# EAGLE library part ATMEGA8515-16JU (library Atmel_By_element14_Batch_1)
Microcontroller with 8K Bytes In-System Programmable Flash
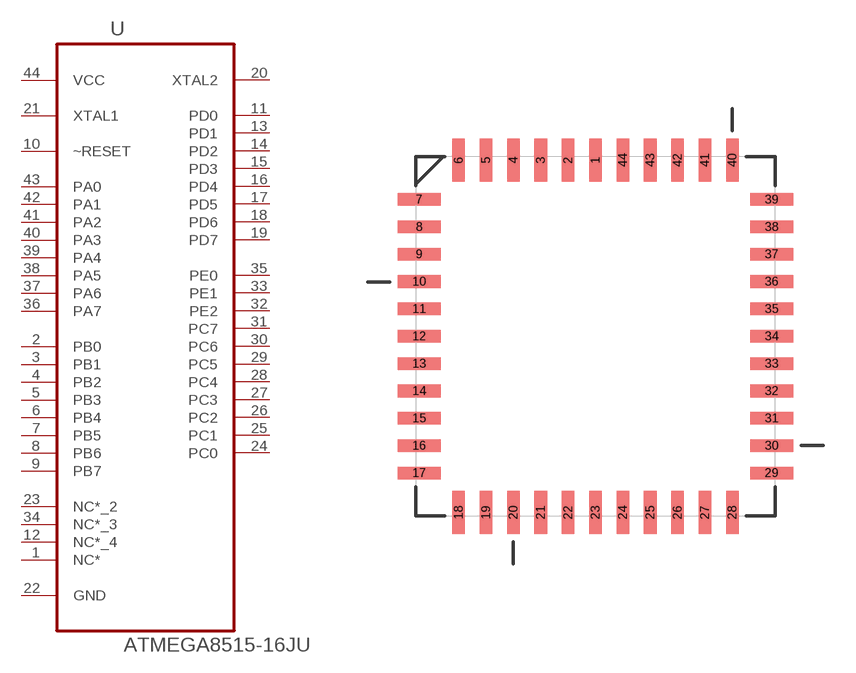
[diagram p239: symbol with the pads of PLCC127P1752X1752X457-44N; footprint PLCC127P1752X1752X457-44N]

Designator prefix U

## ATMEGA8515-16JU (MPN: ATMEGA8515-16JU; OC_FARNELL: 1562624; OC_NEWARK: 94M6261; PACKAGE: PLCC-44; SUPPLIER: Atmel)  [PLCC127P1752X1752X457-44N]
1  NC*  nc
2  PB0
3  PB1
4  PB2
5  PB3
6  PB4
7  PB5
8  PB6
9  PB7
10  ~RESET  in
11  PD0
12  NC*_4  nc
13  PD1
14  PD2
15  PD3
16  PD4
17  PD5
18  PD6
19  PD7
20  XTAL2
21  XTAL1  in
22  GND  pas
23  NC*_2  nc
24  PC0
25  PC1
26  PC2
27  PC3
28  PC4
29  PC5
30  PC6
31  PC7
32  PE2
33  PE1
34  NC*_3  nc
35  PE0
36  PA7
37  PA6
38  PA5
39  PA4
40  PA3
41  PA2
42  PA1
43  PA0
44  VCC  pwr

## Footprint PLCC127P1752X1752X457-44N (pad centres in mm)
smd 0.584 x 2.007: 1 0,8.179; 2 -1.27,8.179; 3 -2.54,8.179; 4 -3.81,8.179; 5 -5.08,8.179; 6 -6.35,8.179; 18 -6.35,-8.179; 19 -5.08,-8.179; 20 -3.81,-8.179; 21 -2.54,-8.179; 22 -1.27,-8.179; 23 0,-8.179; 24 1.27,-8.179; 25 2.54,-8.179; 26 3.81,-8.179; 27 5.08,-8.179; 28 6.35,-8.179; 40 6.35,8.179; 41 5.08,8.179; 42 3.81,8.179; 43 2.54,8.179; 44 1.27,8.179
smd 2.007 x 0.584: 7 -8.179,6.35; 8 -8.179,5.08; 9 -8.179,3.81; 10 -8.179,2.54; 11 -8.179,1.27; 12 -8.179,0; 13 -8.179,-1.27; 14 -8.179,-2.54; 15 -8.179,-3.81; 16 -8.179,-5.08; 17 -8.179,-6.35; 29 8.179,-6.35; 30 8.179,-5.08; 31 8.179,-3.81; 32 8.179,-2.54; 33 8.179,-1.27; 34 8.179,0; 35 8.179,1.27; 36 8.179,2.54; 37 8.179,3.81; 38 8.179,5.08; 39 8.179,6.35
